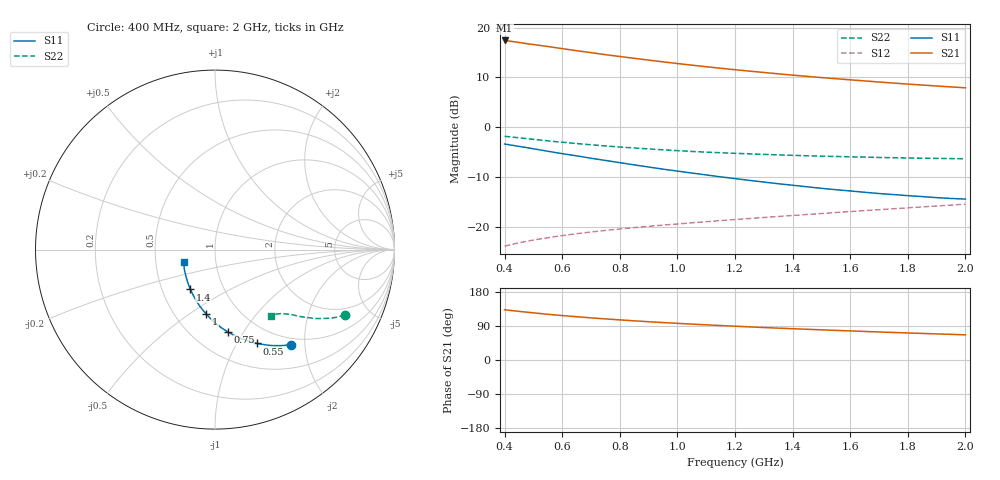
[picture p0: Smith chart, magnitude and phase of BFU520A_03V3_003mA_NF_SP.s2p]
! Filename:  P:\Prog\Test\Noise\ATS_data\Testdata_Net\06 Compressed Noise after Statistics\BFU520A_APG2013_30_A05_03p3V_003mA_NF_CM01_D.sf
! Date/Time: Wed 24/Apr/2013 20:06:16
! BFU520A_APG2013_30_A05_03p3V_1to20mA_NF_CM01_Bias3_R.sf
! Noise Parameter Data File
! BFU520A_APG2013_30_A05_03p3V_1to20mA_NF_CM01
! Date/time: Thu Apr 11 00:04:13 2013
! VAR V_out= 3.300000
! VAR I_out= 3.000000
! VAR V_in= 0.820800
! VAR I_in= 0.033005
! Device data file deembeded for feedlines and parallel
! Original file: \06 Compressed Noise after Statistics\BFU520A_APG2013_30_A05_03p3V_003mA_NF_CM01_R.sf
! Feed-files: PR017V01_150413_Feed1.s2p, PR017V01_150413_Feed2.s2p
! Parallel-file: PR017V01_150413_Par.s2p
# MHz S MA R 50
!  Freq-MHz  S11-mag  S11-arg  S21-mag  S21-arg  S12-mag  S12-arg  S22-mag  S22-arg
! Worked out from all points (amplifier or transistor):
!   37 points, 400 MHz to 2 GHz, reference 50 ohm
!   highest |S21| = 17.4 dB at 400 MHz (marker M1)
!   |S21| within 3 dB of that: start of sweep to 769.5 MHz
!   unconditionally stable (mu >= 1): 1.843 GHz to end of sweep
!   at 500 MHz: K = 0.47, MSG = 19.7 dB, |S12| = -22.7 dB
!   at 1.1 GHz: K = 0.82, MSG = 15.6 dB, |S12| = -19.0 dB
!   at 2 GHz: K = 1.01, MAG = 11.0 dB, |S12| = -15.5 dB
!   lowest NFmin = 0.57 dB at 440 MHz
!   S11 on the Smith chart (normalised r, x): 400 MHz: 0.88, -1.72; 550 MHz: 0.78, -1.22; 750 MHz: 0.73, -0.85; 1 GHz: 0.71, -0.58; 1.4 GHz: 0.69, -0.33; 2 GHz: 0.70, -0.10
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400  0.6772 -51.5  7.447 132.7  0.06366 64.1  0.8101 -26.7
420  0.6626 -53.6  7.315 130.8  0.06578 63.4  0.7987 -27.5
440  0.6485 -55.6  7.181 129.2  0.06783 62.7  0.7875 -28.2
480  0.6213 -59.4  6.896 126.0  0.07157 61.5  0.7651 -29.7
550  0.5733 -65.8  6.478 120.6  0.07741 59.8  0.7286 -31.8
600  0.5417 -70.0  6.165 117.3  0.08131 58.9  0.7059 -33.0
650  0.5151 -73.8  5.872 114.2  0.08497 58.2  0.6851 -34.1
700  0.4877 -77.7  5.618 111.2  0.08834 57.6  0.6656 -35.1
750  0.4632 -81.2  5.361 108.5  0.09164 57.2  0.648 -35.9
800  0.4399 -84.8  5.137 105.9  0.09479 56.9  0.6322 -36.7
850  0.4178 -88.2  4.924 103.4  0.09784 56.6  0.6176 -37.4
900  0.3978 -91.6  4.726 101.0  0.1009 56.5  0.6049 -38.1
950  0.3787 -94.7  4.538 98.8  0.1037 56.5  0.592 -38.7
1000  0.3621 -97.8  4.366 96.7  0.1065 56.5  0.5814 -39.2
1100  0.3312 -104.0  4.054 92.8  0.1122 56.7  0.5617 -40.2
1200  0.3043 -109.9  3.784 89.2  0.1179 56.9  0.546 -41.3
1300  0.281 -115.7  3.55 85.7  0.1237 57.2  0.533 -42.3
1400  0.2608 -121.7  3.338 82.6  0.1296 57.6  0.5217 -43.3
1500  0.2429 -127.7  3.154 79.6  0.1355 58.0  0.5115 -44.2
1650  0.2218 -136.6  2.919 75.3  0.145 58.6  0.5003 -45.8
1750  0.2102 -142.7  2.777 72.6  0.1513 59.0  0.4934 -46.8
2000  0.1893 -157.8  2.489 66.5  0.1683 59.8  0.4816 -49.8
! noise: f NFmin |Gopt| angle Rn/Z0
400  0.6209  0.3744  13.56  0.1633
460  0.6081  0.337  24.11  0.1507
600  0.6916  0.3337  27.44  0.1683
800  0.6598  0.3196  40.5  0.1382
1000  0.6697  0.3072  50.01  0.1343
1200  0.753  0.2877  61.59  0.1259
1400  0.7822  0.2749  73.94  0.1156
1600  0.7791  0.2531  85.19  0.1082
1800  0.7325  0.2533  113.1  0.0807
2000  0.8371  0.2361  116.9  0.0764
